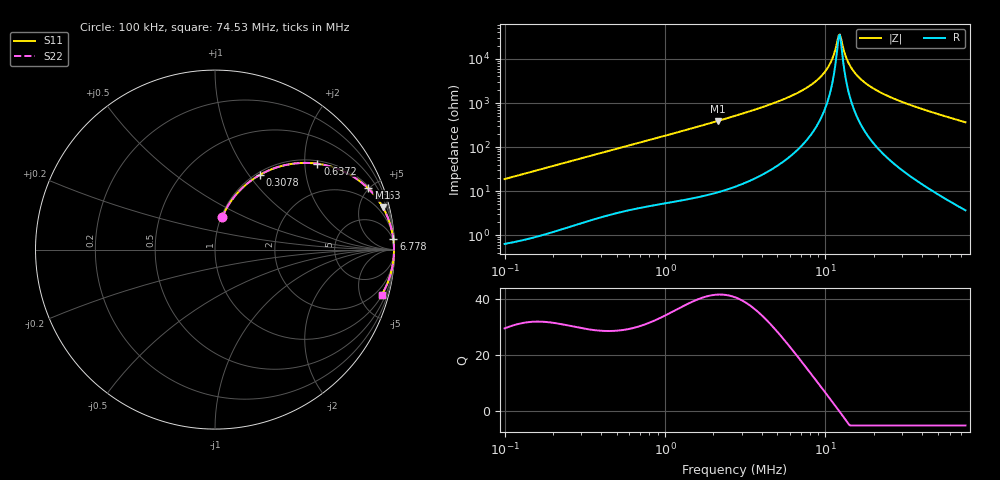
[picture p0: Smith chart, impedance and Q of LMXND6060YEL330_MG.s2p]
! LMXND6060YEL330_MG  S-PARAMETER MODEL  ( General Type )
! Model Generated by TAIYO YUDEN Corporation (https://www.yuden.co.jp/en/)
! Version 1.0
! TAIYO YUDEN Control No. 191025NI43SB-FBB
! Copyright(c) 2019 TAIYO YUDEN CO.,LTD. All Rights Reserved.
! Product Description (link to TY-COMPAS)
! https://ds.yuden.co.jp/TYCOMPAS/or/detail?pn=LMXND6060YEL330MMG&u=M
! Products Name : Inductors
! Characteristics :
!  Inductance : 33 uH , SRF(min) : 6.0 MHz , DC Resistance(max) : 0.1833 Ohm
!  Rated Current : Saturation :1650 mA , Temp Rise : 1400 mA (40 degC)
!  Case Size : 6.0 x 6.0 / 0.236 x 0.236 [mm/inch] , Thickness : 4.5 / 0.177 [mm/inch]
!  (Conditions: Temperature = 25 degC , DC Bias Current/Voltage = 0A / 0V)
! External Node Assignments :
!  1  o---GGG---o  2
! GND o---------o GND
! Frequency Range : 0.1MHz  -  74.526194MHz  [ 402 STEP ]
# MHz S RI R 50
! Freq[MHz].  S11 Real  S11 Imag  S21 Real  S21 Imag  S12 Real  S12 Imag  S22 Real  S22 Imag
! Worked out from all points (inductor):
!   401 points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, 100 kHz to 74.53 MHz, reference 50 ohm
!   read as one part in series: L = 29.8 uH near 103.4 kHz
!   highest Q = 41.7 at 2.13 MHz (marker M1), where L = 29.2 uH
!   self-resonance near 12.09 MHz
!   S11 on the Smith chart (normalised r, x): 100 kHz: 1.01, +0.37; 307.8 kHz: 1.04, +1.14; 637.2 kHz: 1.08, +2.31; 1.363 MHz: 1.13, +4.93; 6.778 MHz: 3, +35; 74.53 MHz: 1.07, -7.31
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0.1  0.0396 0.1789  0.9604 -0.1789  0.9604 -0.1789  0.0396 0.1789
0.181346  0.11 0.2976  0.89 -0.2976  0.89 -0.2976  0.11 0.2976
0.302769  0.2458 0.4141  0.7542 -0.4141  0.7542 -0.4141  0.2458 0.4141
0.307817  0.2516 0.4174  0.7484 -0.4174  0.7484 -0.4174  0.2516 0.4174
0.637157  0.5702 0.4786  0.4298 -0.4786  0.4298 -0.4786  0.5702 0.4786
0.916692  0.7267 0.4308  0.2733 -0.4308  0.2733 -0.4308  0.7267 0.4308
1.363208  0.8522 0.3421  0.1478 -0.3421  0.1478 -0.3421  0.8522 0.3421
2.13031  0.9336 0.2374  0.0664 -0.2374  0.0664 -0.2374  0.9336 0.2374
2.729949  0.9588 0.1869  0.0412 -0.1869  0.0412 -0.1869  0.9588 0.1869
6.777928  0.9937 0.0571  0.00626 -0.0571  0.00626 -0.0571  0.9937 0.0571
8.265445  0.9958 0.0368  0.00422 -0.0368  0.00422 -0.0368  0.9958 0.0368
9.434359  0.9966 0.024  0.00339 -0.024  0.00339 -0.024  0.9966 0.024
10.4183  0.997 0.0147  0.00299 -0.0147  0.00299 -0.0147  0.997 0.0147
11.13064  0.9972 0.00863  0.00283 -0.00863  0.00283 -0.00863  0.9972 0.00863
11.89168  0.9973 0.00256  0.00275 -0.00256  0.00275 -0.00256  0.9973 0.00256
12.2915  0.9973 -0.000475  0.00273 0.000475  0.00273 0.000475  0.9973 -0.000475
12.49642  0.9973 -0.00199  0.00273 0.00199  0.00273 0.00199  0.9973 -0.00199
13.79972  0.9972 -0.0111  0.00283 0.0111  0.00283 0.0111  0.9972 -0.0111
15.493  0.9968 -0.0219  0.00317 0.0219  0.00317 0.0219  0.9968 -0.0219
18.89317  0.9956 -0.0411  0.00437 0.0411  0.00437 0.0411  0.9956 -0.0411
25.02522  0.9923 -0.0711  0.00775 0.0711  0.00775 0.0711  0.9923 -0.0711
74.52619  0.9283 -0.2531  0.0717 0.2531  0.0717 0.2531  0.9283 -0.2531
